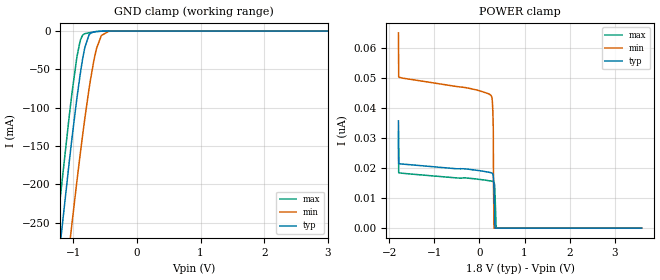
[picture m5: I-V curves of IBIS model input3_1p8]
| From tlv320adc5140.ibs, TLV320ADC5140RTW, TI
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|   input3_1p8 Model
[Model]   input3_1p8
Model_type   Input
Vinl = 0.63
Vinh = 1.17
|   typ   min   max
C_comp   1.6056pF   1.5123pF   1.7126pF
[Model spec]
|subparameter
Vinl   0.63   0.567   0.693
Vinh   1.17   1.053   1.287
| Where Nom  PVT is Nominal Process, 1.8V, 27C
|   Fast PVT is Strong Process,  1.98V, -40C
|   Slow PVT is Weak Process,   1.62V, 150C
[Voltage Range]   1.8   1.62   1.98
|Junction Temperature
[Temperature Range]   27   150   -40
[Power Clamp Reference]   1.8   1.62   1.98
[GND Clamp Reference]   0   0   0
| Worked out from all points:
|   GND clamp passes 1 mA (typ) near -0.68 V on its own axis
[GND Clamp]
|   Voltage   I(typ)   I(min)   I(max)
-1.8V     -769.5mA   -875.2mA   -713.7mA
-1.465V   -489.3mA   -598.8mA   -430.9mA
-1.228V   -297.1mA   -409.1mA   -236.9mA
-1.206V   -280.1mA   -392.2mA   -219.8mA
-1.028V   -146.1mA   -257.6mA   -86.97mA
-892.8mV  -58.14mA   -162.8mA   -13.66mA
-817.2mV  -21.44mA   -114.2mA   -3.411mA
-747mV    -4.516mA   -73.4mA    -2.142mA
-633.6mV  -501.4uA   -22.73mA   -687.9uA
-558mV    -123.2uA   -5.762mA   -167.6uA
-444.6mV  -3.833uA   -359.9uA   -2.902uA
3.6V      0A         0A         0A
[POWER Clamp]
|   Voltage   I(typ)   I(min)   I(max)
-1.8V     35.63nA    64.89nA    32.03nA
-1.795V   21.46nA    50.3nA     18.4nA
-1.789V   21.43nA    50.22nA    18.38nA
262.8mV   18.39nA    43.91nA    15.65nA
289.8mV   18.1nA     40.98nA    15.54nA
306mV     17.26nA    33.1nA     15.47nA
311.4mV   16.35nA    13.99nA    15.41nA
322.2mV   12.57nA    0A         15.2nA
338.4mV   1.81nA     0A         13.6nA
365.4mV   0A         0A         1.347nA
376.2mV   0A         0A         0A
3.6V      0A         0A         0A
